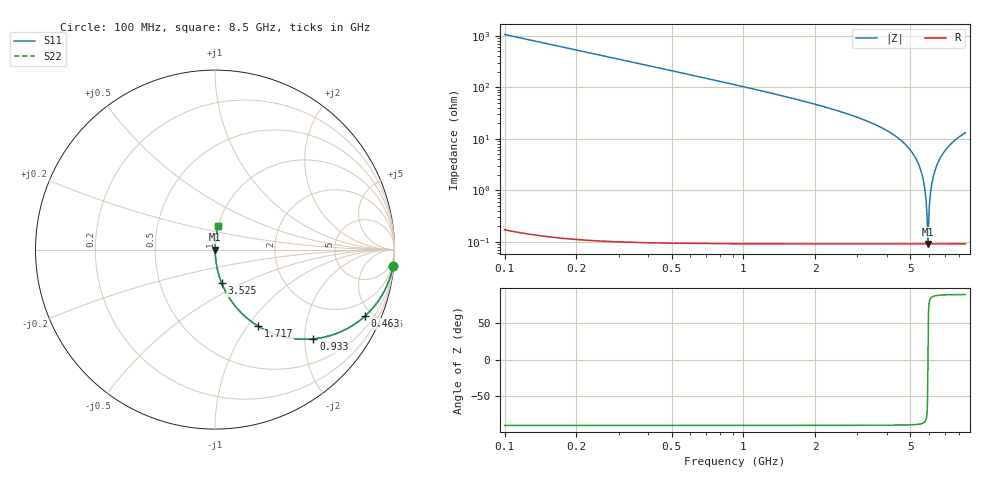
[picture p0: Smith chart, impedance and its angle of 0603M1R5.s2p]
! Created Wed Apr 18 13:47:23 2012
# hz S ma R 50
! 2 Port Network Data from SP1.SP block
! freq  magS11  angS11  magS21  angS21  magS12  angS12  magS22  angS22
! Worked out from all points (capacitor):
!   8401 points, 100 MHz to 8.5 GHz, reference 50 ohm
!   read as one part in series: C = 1.51 pF near 142 MHz
!   lowest |Z| = 91.9 mohm at 5.923 GHz (marker M1)
!   series resonance near 5.923 GHz, so ESL is about 480 pH
!   S11 on the Smith chart (normalised r, x): 100 MHz: 1, -21; 463 MHz: 1.00, -4.53; 933 MHz: 1.00, -2.20; 1.717 GHz: 1.00, -1.12; 3.525 GHz: 1.00, -0.39; 8.5 GHz: 1.00, +0.26
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1e8  0.9955 -5.4  0.09448 84.6  0.09448 84.6  0.9955 -5.4
2.56e8  0.9716 -13.7  0.2364 76.3  0.2364 76.3  0.9716 -13.7
4.63e8  0.9145 -23.8  0.4042 66.1  0.4042 66.1  0.9145 -23.8
9.33e8  0.7401 -42.2  0.6718 47.7  0.6718 47.7  0.7401 -42.2
1.5e9  0.5491 -56.6  0.835 33.3  0.835 33.3  0.5491 -56.6
1.717e9  0.4898 -60.6  0.871 29.3  0.871 29.3  0.4898 -60.6
2.9e9  0.2661 -74.4  0.963 15.4  0.963 15.4  0.2661 -74.4
3.525e9  0.1895 -78.8  0.981 10.9  0.981 10.9  0.1895 -78.8
4.3e9  0.1151 -82.9  0.9924 6.6  0.9924 6.6  0.1151 -82.9
5.222e9  0.04487 -86.3  0.9981 2.6  0.9981 2.6  0.04487 -86.3
5.506e9  0.02598 -86.5  0.9987 1.5  0.9987 1.5  0.02598 -86.5
5.7e9  0.01366 -85.4  0.999 0.8  0.999 0.8  0.01366 -85.4
5.816e9  0.006526 -81.5  0.9991 0.4  0.9991 0.4  0.006526 -81.5
5.897e9  0.001792 -59.1  0.9991 0.1  0.9991 0.1  0.001792 -59.1
5.923e9  0.0009183 1.7  0.9991 -0.0  0.9991 -0.0  0.0009183 1.7
5.947e9  0.001729 57.9  0.9991 -0.1  0.9991 -0.1  0.001729 57.9
5.998e9  0.004597 78.2  0.9991 -0.3  0.9991 -0.3  0.004597 78.2
6.05e9  0.007632 82.7  0.9991 -0.4  0.9991 -0.4  0.007632 82.7
6.231e9  0.0181 86.1  0.9989 -1.0  0.9989 -1.0  0.0181 86.1
6.57e9  0.03698 86.5  0.9984 -2.1  0.9984 -2.1  0.03698 86.5
7.1e9  0.06477 85.5  0.997 -3.7  0.997 -3.7  0.06477 85.5
8.5e9  0.1304 82.1  0.9906 -7.5  0.9906 -7.5  0.1304 82.1
